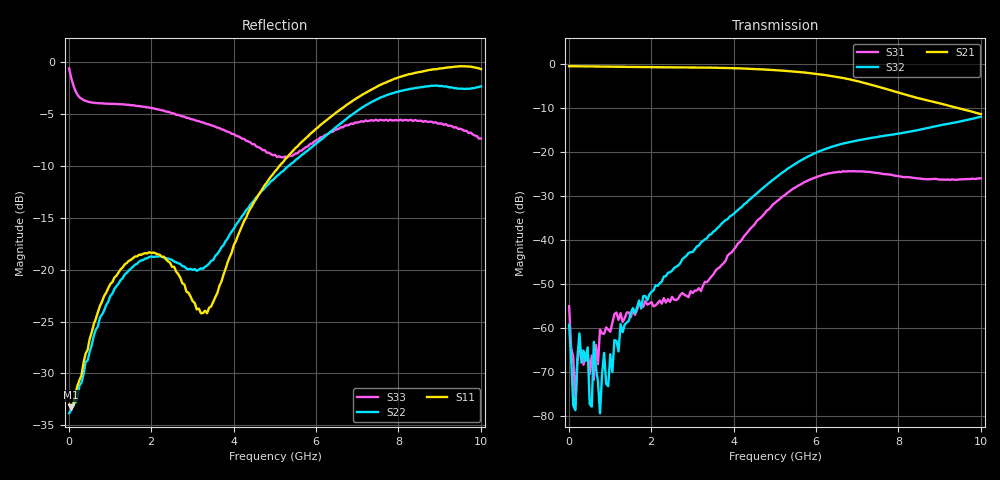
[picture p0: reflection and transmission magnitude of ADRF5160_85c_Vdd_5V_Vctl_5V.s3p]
! Device:  ADRF5160
! Description: Silicon SPDT Switch
! Frequency:  0.7 -  4 GHz
! Ports:
!	RFc	= Port 1
!	RF1	= Port 2
!  RF2  = Port 3
! Vdd:  5 Volt
! Control:  5 Volt
! Data:  Data was collected using a calibrated 4 port network analyzer and de-embedded using Agilent's AFR De-Embedding.
! Note:  Analog Devices supplies this data as a sample of measured data
!  for this product.  Your particular data for this product may vary.
!  Data was taken at 85 degrees C.
!S3P File: Measurements: <S11,S12,S13>,
!<S21,S22,S23>,
!<S31,S32,S33>:
# Hz S  dB  R 50
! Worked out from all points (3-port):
!   201 points, 10 MHz to 10 GHz, reference 50 ohm
!   strongest paths, dB at 10 MHz, 2.507 GHz, 5.005 GHz, 7.503 GHz, 10 GHz:
!     S21: -0.5, -0.8, -1.4, -5.2, -11.4
!     S32: -59.3, -47.0, -26.0, -16.6, -12.0
!     S31: -55.1, -52.9, -31.6, -24.8, -26.0
!   lowest |S11| = -33.3 dB at 59.95 MHz (marker M1), VSWR 1.04, Z = 52.1 - j0.814 ohm
!   |S11| at or under -10 dB: start of sweep to 5.117 GHz
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1e7  -33.00 -18.3  -0.48 0.0  -51.40 -49.5
     -0.52 -0.5  -33.84 -18.5  -63.90 38.4
     -55.05 1.4  -59.30 -105.7  -0.63 -8.9
5.995e7  -33.26 -21.1  -0.55 -1.7  -66.32 -157.4
         -0.52 -1.7  -33.51 -18.2  -69.02 164.4
         -64.58 113.5  -67.08 79.2  -1.53 -45.2
1.5985e8  -31.98 -39.0  -0.54 -4.4  -68.49 36.8
          -0.55 -4.4  -32.84 -38.6  -73.68 49.5
          -78.23 106.2  -78.67 38.0  -2.76 -94.2
2.5975e8  -30.65 -55.1  -0.55 -7.0  -71.79 99.8
          -0.55 -7.0  -31.18 -54.3  -64.54 84.1
          -65.39 -152.1  -61.22 32.2  -3.41 -122.2
3.5965e8  -28.97 -62.1  -0.56 -9.7  -69.69 69.0
          -0.57 -9.7  -30.12 -63.6  -88.15 174.1
          -68.34 50.4  -65.16 -32.9  -3.68 -139.2
4.096e8  -28.11 -68.5  -0.56 -11.0  -73.46 62.5
         -0.56 -11.0  -28.91 -70.1  -63.40 30.5
         -65.91 23.9  -67.50 42.3  -3.76 -145.4
6.5935e8  -24.73 -84.1  -0.58 -17.6  -65.05 62.0
          -0.58 -17.6  -25.76 -91.9  -69.78 -19.7
          -63.88 87.4  -68.95 -54.2  -3.96 -165.3
7.5925e8  -23.50 -88.0  -0.60 -20.3  -60.28 68.1
          -0.60 -20.3  -24.60 -99.8  -71.02 -156.0
          -60.34 54.2  -79.39 70.0  -3.99 -170.6
5.005e9  -10.54 17.0  -1.42 -138.5  -31.60 100.9
         -1.43 -138.5  -11.17 -121.9  -26.01 118.5
         -31.58 100.1  -25.97 118.9  -8.95 105.0
1e10  -0.69 -84.4  -11.41 87.0  -25.91 -87.4
      -11.40 86.9  -2.35 79.8  -11.99 -74.2
      -26.00 -87.4  -11.99 -74.2  -7.38 8.0
